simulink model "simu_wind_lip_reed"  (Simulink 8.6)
settings: Solver=ode4  StartTime=0.0  StopTime=runtime  FixedStep=1/fs  RelTol=1e-3
PostLoadFcn:
  | , if any(exist('dsrtsu_mdlpostloadfcn', 'file') == [2, 3, 6]), try dsrtsu_mdlpostloadfcn('Execute', bdroot); catch fprintf('Error in PostLoadFcn (dsrtsu_mdlpostloadfcn) for model "%s":
  |  %s
  | ', bdroot, lasterr); end, end,
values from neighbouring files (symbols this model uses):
  ae = 1.5 gives smoother results, so more realistic, but it destabilises the hybrid instrument!    [lip_reed.m]
  alpha_Qr = alpha_wr/alpha_r    [lip_reed.m]
  alpha_wr = sqrt(alpha_k)    [lip_reed.m]
  an = modal_coeff(:,1)    [hybrid_wind.m]
  gammal_cte = 2    [lip_reed.m]
  PM = 50    [bowed_string_hyperbolic.m]    (also in lip_reed.m = 20; single_reed.m = 100)
  Qn = modal_coeff(:,3)    [hybrid_wind.m]
  Qr = 3    [lip_reed.m]    (also in single_reed.m = 5)
  Ts = 25e-6    (= 2.5e-05)    [hybrid_wind.m]    (also in measurements.m)
  wn = modal_coeff(:,2)    [hybrid_wind.m]
  wr = 2*pi*140*0.7    (= 615.752160104)    [lip_reed.m]    (also in single_reed.m = 15707.9632679)
  yb = 1    [lip_reed.m]
  yth = yb+0.2    (= 1.2)    [lip_reed.m]
  Zc = rho*c/St    (= 2615281.00417)    [hybrid_wind.m]
  zetal = 0.15    [lip_reed.m]
undefined symbols (not defined in the file or in its folder): modal_coeff, sigbuilder_block
libraries: simulink x1

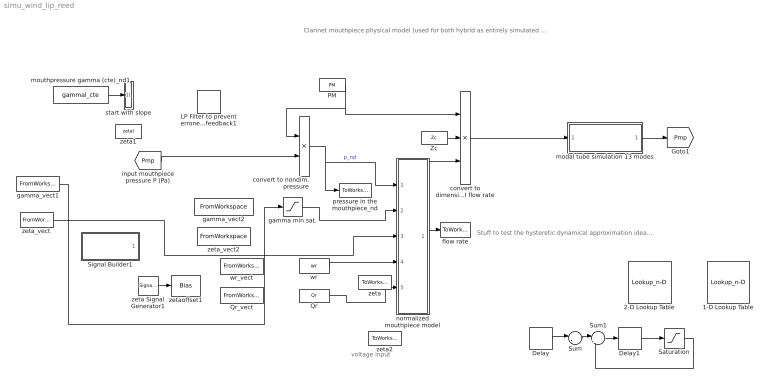
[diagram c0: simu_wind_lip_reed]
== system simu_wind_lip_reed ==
  note: Stuff to test the hysteretic dynamical approximation idea...
  note: Clarinet mouthpiece physical model (used for both hybrid as entirely simulated clarinets)
  note: voltage input
  1-D Lookup Table : Lookup_n-D  NumberOfTableDimensions=1  BreakpointsForDimension1=[-5:5]  BreakpointsForDimension1FirstPoint=10  BreakpointsForDimension2FirstPoint=10  BreakpointsForDimension1Spacing=12  BreakpointsForDimension2Spacing=12  IndexSearchMethod=Evenly spaced points  Table=tanh([-5:5])  InterpMethod=Flat  DiagnosticForOutOfRangeInput=Error  InternalRulePriority=Speed  RndMeth=Simplest
  2-D Lookup Table : Lookup_n-D  BreakpointsForDimension1=[1:3]  BreakpointsForDimension2=[1:3]  InternalRulePriority=Speed  RndMeth=Simplest
  Delay : Delay  DelayLength=1  InitialCondition=0
  Delay1 : Delay  DelayLength=1  InitialCondition=0
  LP Filter to prevent erroneous high freq feedback1 : DiscreteFilter  Numerator=HdLP.ScaleValues(1)*HdLP.sosMatrix(1:end/2)  Denominator=HdLP.ScaleValues(2)*HdLP.sosMatrix(1+end/2:end)  SampleTime=Ts
  PM : Constant  Value=PM
  Qr : Constant  Value=Qr
  Qr_vect : FromWorkspace  VariableName=Qr_vect  SampleTime=0  OutputAfterFinalValue=Setting to zero
  Saturation : Saturate
  Signal Builder1 : Subsystem  Tag=STV Subsys  LoadFcn=sigbuilder_block('load');  StartFcn=sigbuilder_block('start');  StopFcn=sigbuilder_block('stop');  ClipboardFcn=sigbuilder_block('clipboard');
  Sum : Sum  Inputs=|-+
  Sum1 : Sum  Inputs=|+-
  Zc : Constant  Value=Zc
  convert to dimensional flow rate : Product  Inputs=*/*
  convert to nondim. pressure : Product  Inputs=/*
  flow rate : ToWorkspace  VariableName=q_dl  SaveFormat=Structure  SampleTime=-1
  gamma min sat. : Saturate  UpperLimit=100  LowerLimit=0.3
  gamma_vect1 : FromWorkspace  VariableName=gammal_vect  SampleTime=0  OutputAfterFinalValue=Setting to zero
  gamma_vect2 : FromWorkspace  VariableName=gammal_envs_all  SampleTime=0
  modal tube simulation 13 modes : Subsystem
  mouthpressure gamma (cte)_nd1 : Constant  Value=gammal_cte
  normalized mouthpiece model : Subsystem
  pressure in the mouthpiece_nd : ToWorkspace  VariableName=p_dl  SaveFormat=Structure  SampleTime=-1
  start with slope : Subsystem
  wr : Constant  Value=wr
  wr_vect : FromWorkspace  VariableName=wr_vect  SampleTime=0  OutputAfterFinalValue=Setting to zero
  zeta : ToWorkspace  VariableName=wr_vect_simu  SaveFormat=Structure  SampleTime=-1
  zeta Signal Generator1 : SignalGenerator  WaveForm=sawtooth  Amplitude=(0.6-0.1)/2  Frequency=0.2
  zeta1 : Constant  Value=zetal
  zeta2 : ToWorkspace  VariableName=Qr_vect_simu  SaveFormat=Structure  SampleTime=-1
  zeta_vect : FromWorkspace  VariableName=zetal_vect  SampleTime=0  OutputAfterFinalValue=Setting to zero
  zeta_vect2 : FromWorkspace  VariableName=zetal_envs_all  SampleTime=0  OutputAfterFinalValue=Setting to zero
  zetaoffset1 : Bias  Bias=0.1+(0.6-0.1)/2
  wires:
  modal tube simulation 13 modes/1(p_sim_out) -> [Pmp]
  zeta Signal Generator1/1 -> zetaoffset1/1
  Zc/1 -> convert to dimensional flow rate/2
  convert to nondim. pressure/1 -> normalized mouthpiece model/1(p), pressure in the mouthpiece_nd/1  "p_nd"
  PM/1 -> convert to nondim. pressure/1, convert to dimensional flow rate/1
  normalized mouthpiece model/1(u_nd) -> flow rate/1, convert to dimensional flow rate/3
  convert to dimensional flow rate/1 -> modal tube simulation 13 modes/1(flowrate_in)
  [Pmp] -> convert to nondim. pressure/2
  wr/1 -> normalized mouthpiece model/4(wr)
  Qr/1 -> normalized mouthpiece model/5(Qr)
  ? -> Sum/2, Delay/1
  Delay/1 -> Sum/1
  Sum/1 -> Sum1/1
  Sum1/1 -> Delay1/1
  Delay1/1 -> Saturation/1
  Saturation/1 -> Sum1/2
  mouthpressure gamma (cte)_nd1/1 -> start with slope/1(gamma_in)
  gamma min sat./1 -> normalized mouthpiece model/2(gamma)
  zeta_vect/1 -> normalized mouthpiece model/3(zeta)
  gamma_vect1/1 -> gamma min sat./1

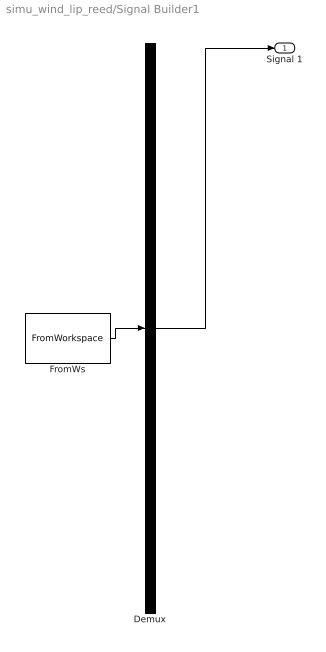
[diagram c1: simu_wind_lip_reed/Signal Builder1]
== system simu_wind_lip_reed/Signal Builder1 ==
  Demux : Demux  Tag=STV Demux  Outputs=1
  FromWs : FromWorkspace  Tag=STV FromWs  VariableName=tuvar  SampleTime=0  SigBuilderData=DataTag0  VnvData=DataTag1
  Signal 1 : Outport  Tag=STV Outport
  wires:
  Demux/1 -> Signal 1/1
  FromWs/1 -> Demux/1

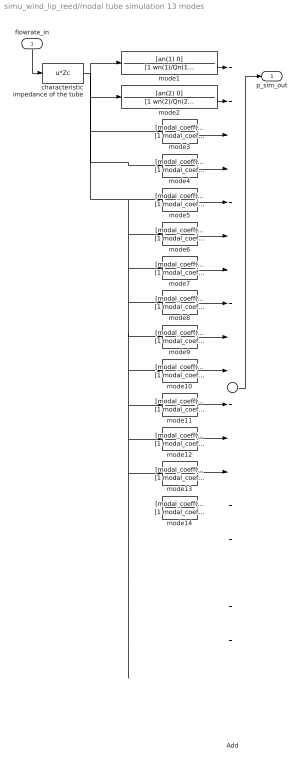
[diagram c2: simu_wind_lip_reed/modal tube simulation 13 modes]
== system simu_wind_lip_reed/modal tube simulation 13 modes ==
  flowrate_in : Inport
  Add : Sum  Inputs=++++++++++++++++++++
  characteristic impedance of the tube : Fcn  Expr=u*Zc
  mode1 : TransferFcn  Numerator=[an(1) 0]  Denominator=[1 wn(1)/Qn(1) wn(1)^2]
  mode10 : TransferFcn  Numerator=[modal_coeff(10, 1) 0]  Denominator=[1 modal_coeff(10,2)/modal_coeff(10,3) modal_coeff(10,2)^2]
  mode11 : TransferFcn  Numerator=[modal_coeff(11, 1) 0]  Denominator=[1 modal_coeff(11,2)/modal_coeff(11,3) modal_coeff(11,2)^2]
  mode12 : TransferFcn  Numerator=[modal_coeff(12, 1) 0]  Denominator=[1 modal_coeff(12,2)/modal_coeff(12,3) modal_coeff(12,2)^2]
  mode13 : TransferFcn  Numerator=[modal_coeff(13, 1) 0]  Denominator=[1 modal_coeff(13,2)/modal_coeff(13,3) modal_coeff(13,2)^2]
  mode14 : TransferFcn  Numerator=[modal_coeff(14, 1) 0]  Denominator=[1 modal_coeff(14,2)/modal_coeff(14,3) modal_coeff(14,2)^2]
  mode2 : TransferFcn  Numerator=[an(2) 0]  Denominator=[1 wn(2)/Qn(2) wn(2)^2]
  mode3 : TransferFcn  Numerator=[modal_coeff(3, 1) 0]  Denominator=[1 modal_coeff(3,2)/modal_coeff(3,3) modal_coeff(3,2)^2]
  mode4 : TransferFcn  Numerator=[modal_coeff(4, 1) 0]  Denominator=[1 modal_coeff(4,2)/modal_coeff(4,3) modal_coeff(4,2)^2]
  mode5 : TransferFcn  Numerator=[modal_coeff(5, 1) 0]  Denominator=[1 modal_coeff(5,2)/modal_coeff(5,3) modal_coeff(5,2)^2]
  mode6 : TransferFcn  Numerator=[modal_coeff(6, 1) 0]  Denominator=[1 modal_coeff(6,2)/modal_coeff(6,3) modal_coeff(6,2)^2]
  mode7 : TransferFcn  Numerator=[modal_coeff(7, 1) 0]  Denominator=[1 modal_coeff(7,2)/modal_coeff(7,3) modal_coeff(7,2)^2]
  mode8 : TransferFcn  Numerator=[modal_coeff(8, 1) 0]  Denominator=[1 modal_coeff(8,2)/modal_coeff(8,3) modal_coeff(8,2)^2]
  mode9 : TransferFcn  Numerator=[modal_coeff(9, 1) 0]  Denominator=[1 modal_coeff(9,2)/modal_coeff(9,3) modal_coeff(9,2)^2]
  p_sim_out : Outport
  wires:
  flowrate_in/1 -> characteristic impedance of the tube/1
  characteristic impedance of the tube/1 -> mode4/1, mode3/1, mode2/1, mode1/1, mode5/1, mode6/1, mode7/1, mode8/1, mode9/1, mode10/1, mode11/1, mode12/1, mode13/1
  mode1/1 -> Add/1
  Add/1 -> p_sim_out/1
  mode2/1 -> Add/2
  mode3/1 -> Add/3
  mode4/1 -> Add/4
  mode5/1 -> Add/5
  mode6/1 -> Add/6
  mode7/1 -> Add/7
  mode8/1 -> Add/8
  mode9/1 -> Add/9
  mode10/1 -> Add/10
  mode11/1 -> Add/11
  mode12/1 -> Add/12
  mode13/1 -> Add/13
  ? -> Add/15

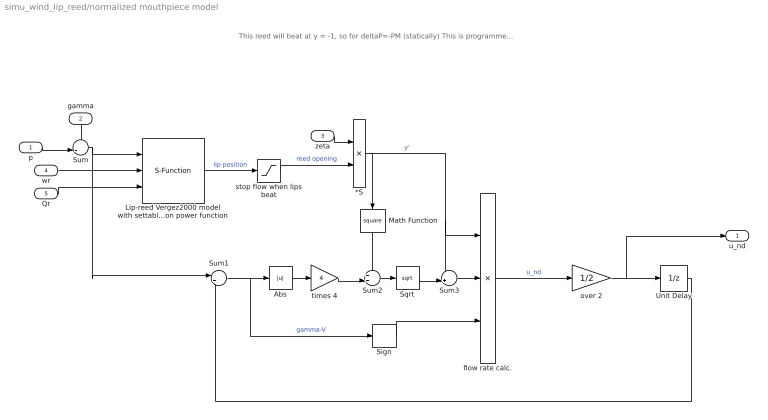
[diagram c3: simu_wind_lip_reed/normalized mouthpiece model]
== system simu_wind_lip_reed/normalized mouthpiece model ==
  note: This reed will beat at y = -1, so for deltaP=-PM (statically) This is programmed in the LP filter, which switches coefficients.
  p : Inport
  gamma : Inport  Port=2
  zeta : Inport  Port=3
  wr : Inport  Port=4
  Qr : Inport  Port=5
  *S : Product  Inputs=**
  Abs : Abs
  Lip-reed Vergez2000 model with settable rest-position offset and opening section power function : S-Function  InitFcn=try, set_param(gcb,'FunctionName','reed_discrete_LP_filter_hitting_reed'), end  FunctionName=reed_discrete_LP_filter_hitting_reed  Parameters=1/Ts,alpha_wr,alpha_Qr,yth,yb,ae  SFunctionModules=reed_discrete_LP_filter_hitting_reed_wrapper  WizardData=DataTag2  SFunctionDeploymentMode=off  EnableBusSupport=off
  Math Function : Math  Operator=square
  Sign : Signum
  Sqrt : Sqrt
  Sum : Sum  Inputs=+-|
  Sum1 : Sum  Inputs=|++
  Sum2 : Sum  Inputs=++|
  Sum3 : Sum  Inputs=-+|
  Unit Delay : UnitDelay  SampleTime=-1
  flow rate calc. : Product  Inputs=3
  over 2 : Gain  Gain=1/2
  stop flow when lips beat : Saturate  UpperLimit=100  LowerLimit=0
  times 4 : Gain  Gain=4
  u_nd : Outport
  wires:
  zeta/1 -> *S/1
  Sum2/1 -> Sqrt/1
  Sum1/1 -> Abs/1, Sign/1  "gamma-V"
  Sum/1 -> Sum1/1, Lip-reed Vergez2000 model with settable rest-position offset and opening section power function/1
  *S/1 -> flow rate calc./1, Sum3/1, Math Function/1  "y'"
  flow rate calc./1 -> over 2/1  "u_nd"
  Sqrt/1 -> Sum3/2
  Sum3/1 -> flow rate calc./2
  over 2/1 -> u_nd/1, Unit Delay/1
  Math Function/1 -> Sum2/1
  Abs/1 -> times 4/1
  times 4/1 -> Sum2/2
  Sign/1 -> flow rate calc./3
  Unit Delay/1 -> Sum1/2
  wr/1 -> Lip-reed Vergez2000 model with settable rest-position offset and opening section power function/2
  Qr/1 -> Lip-reed Vergez2000 model with settable rest-position offset and opening section power function/3
  gamma/1 -> Sum/1
  Lip-reed Vergez2000 model with settable rest-position offset and opening section power function/1 -> stop flow when lips beat/1  "lip position"
  p/1 -> Sum/2
  stop flow when lips beat/1 -> *S/2  "reed opening"

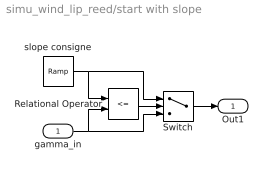
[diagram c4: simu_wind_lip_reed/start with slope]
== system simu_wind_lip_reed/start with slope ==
  gamma_in : Inport
  Relational Operator : RelationalOperator  Operator=<=  OutDataTypeStr=boolean
  Switch : Switch  Criteria=u2 > Threshold
  slope consigne : simulink/Sources/Ramp  slope=gammal_cte*100  start=0  X0=0
  Out1 : Outport
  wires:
  slope consigne/1 -> Relational Operator/1, Switch/1
  gamma_in/1 -> Relational Operator/2, Switch/3
  Relational Operator/1 -> Switch/2
  Switch/1 -> Out1/1
